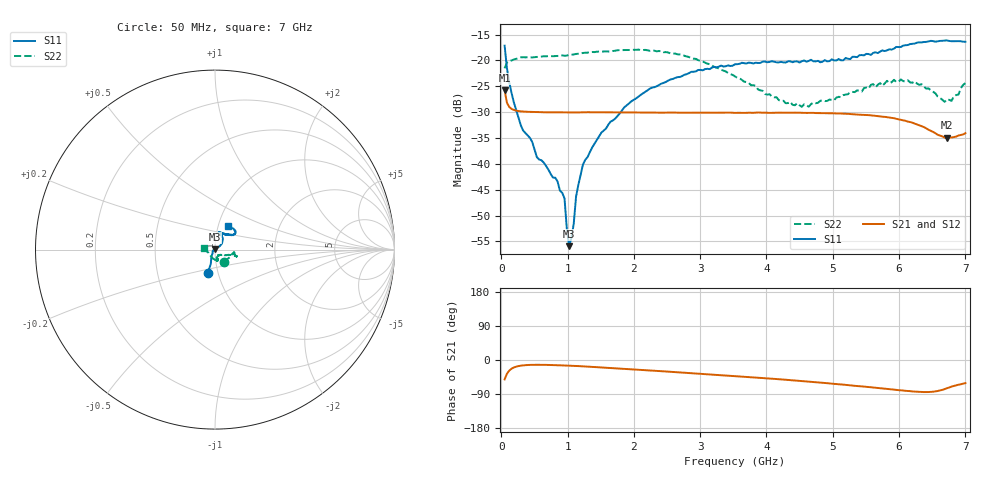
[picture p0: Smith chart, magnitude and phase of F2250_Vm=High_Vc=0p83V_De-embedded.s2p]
! Integrated Device Technology
! Corporate Headquarters
! 6024 Silver Creek Valley Road
! San Jose, CA 95138  USA
! Phone:  1-408-284-8200
! Toll Free:  1-800-223-1366
! Webpage:  http://www.idt.com/
! Timing and RF Division
! 515 Groton Road, Suite 102
! Westford, MA 01886-6024
! Device:  F2250
! Description: Voltage Variable RF Attenuator
! Frequency:  50.0 -  6000.00 MHz
! Package:  3x3 mm Thin QFN Plastic Package: 16 pin
! Ports:  2 RF, 3 DC
!  Pin  1  = GND
!  Pin  2  = NC
!  Pin  3  = RF1  = Port 1
!  Pin  4  = NC
!  Pin  5  = GND
!  Pin  6  = GND
!  Pin  7  = GND
!  Pin  8  = GND
!  Pin  9  = NC
!  Pin 10  = RF2  = Port 2
!  Pin 11  = NC
!  Pin 12  = GND
!  Pin 13  = GND
!  Pin 14  = VCNTRL
!  Pin 15  = VDD
!  Pin 16  = VMODE
! Vcntrl:  0.830 Volts
! Vmode:  +3.300 Volts
! Vdd:  +3.30  Volts
! Current:  1.307 mA
! Data:  The device was measured on a the F2250 evaluation board which has
!  individual transmission lines to the RF pins.  Data was collected
!  using a calibrated network analyzer.  The evaluation board was
!  de-embedded using a TRL calibration technique.
!  The reference plane is the edge of the package pin.
! Misc:  SN 10
!  Action Tracker AT0258
! Date Measured:  2014-11-26
! Date:  2015-10-15  MJV
! Note:
!  Integrated Device Technology supplies this data as a sample of measured
!  data at the package pin for this product.  Your particular data for this
!  product may vary.
!  Data was taken at 25 degrees C.
!  Integrated Device Technology reserves the right to change this data at anytime.
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# GHz S dB R 50
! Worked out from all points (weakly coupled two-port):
!   201 points, 50 MHz to 7 GHz, reference 50 ohm
!   highest |S21| = -25.79 dB at 50 MHz (marker M1); lowest = -34.9 dB at 6.722 GHz (marker M2)
!   lowest |S11| = -55.9 dB at 1.023 GHz (marker M3), VSWR 1.00, Z = 49.9 + j0.136 ohm
!   |S11| at or under -10 dB: start of sweep to end of sweep
!   |S22| runs from -29.0 to -17.9 dB; largest |S21 - S12| = 0.00011
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0.05  -17.15 -107.5  -25.79 -51.2  -25.79 -51.2  -21.54 -53.7
0.1195  -24.22 -110.4  -29.01 -28.0  -29.00 -28.0  -20.15 -15.6
0.29325  -32.50 -124.1  -29.85 -15.0  -29.83 -15.0  -19.42 -9.4
0.467  -35.79 -142.2  -29.97 -12.8  -29.95 -12.8  -19.43 -8.0
0.5365  -38.71 -149.8  -29.98 -12.6  -29.98 -12.7  -19.33 -8.9
0.8145  -42.69 171.3  -30.05 -13.6  -30.03 -13.6  -19.17 -11.8
0.9535  -46.68 174.6  -30.05 -14.4  -30.04 -14.5  -19.11 -13.4
0.98825  -52.52 168.7  -30.04 -14.7  -30.06 -14.7  -19.06 -13.7
1.023  -55.92 121.4  -30.06 -14.9  -30.07 -14.9  -18.95 -13.7
1.0925  -51.62 56.0  -30.06 -15.4  -30.04 -15.5  -18.86 -14.2
1.12725  -46.40 43.6  -30.06 -15.7  -30.05 -15.7  -18.76 -14.7
1.2315  -40.16 32.7  -30.02 -16.7  -30.03 -16.7  -18.56 -16.1
1.6485  -31.85 38.0  -30.03 -21.1  -30.04 -21.1  -18.24 -17.2
2.37825  -24.74 45.2  -30.10 -29.2  -30.12 -29.1  -18.19 -17.5
3.525  -20.74 71.0  -30.15 -42.4  -30.13 -42.5  -23.09 -26.2
4.2895  -20.41 75.3  -30.11 -52.1  -30.12 -52.1  -28.28 -50.2
4.7065  -20.17 71.5  -30.15 -58.1  -30.16 -58.1  -28.17 -68.5
5.85325  -17.85 40.1  -31.06 -77.0  -31.04 -77.1  -24.42 -76.5
6.2355  -16.75 38.6  -32.23 -83.4  -32.21 -83.4  -24.05 -85.0
6.722  -16.15 49.0  -34.95 -74.4  -34.94 -74.5  -27.52 -143.9
6.7915  -16.30 51.0  -34.91 -70.2  -34.94 -70.2  -27.83 -157.5
7  -16.41 62.0  -34.07 -61.2  -34.04 -61.4  -24.40 172.8
